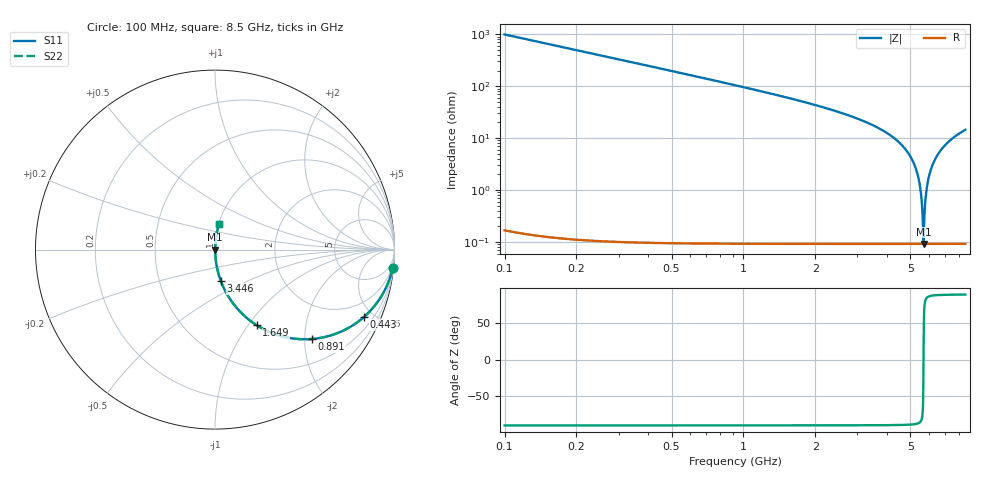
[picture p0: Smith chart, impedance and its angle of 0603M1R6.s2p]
! Created Wed Apr 18 13:49:44 2012
# hz S ma R 50
! 2 Port Network Data from SP1.SP block
! freq  magS11  angS11  magS21  angS21  magS12  angS12  magS22  angS22
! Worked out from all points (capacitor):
!   8401 points, 100 MHz to 8.5 GHz, reference 50 ohm
!   read as one part in series: C = 1.61 pF near 142 MHz
!   lowest |Z| = 92 mohm at 5.677 GHz (marker M1)
!   series resonance near 5.677 GHz, so ESL is about 490 pH
!   S11 on the Smith chart (normalised r, x): 100 MHz: 1, -20; 443 MHz: 1.00, -4.44; 891 MHz: 1.00, -2.16; 1.649 GHz: 1.00, -1.10; 3.446 GHz: 1.00, -0.36; 8.5 GHz: 1.00, +0.29
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1e8  0.9949 -5.8  0.1007 84.2  0.1007 84.2  0.9949 -5.8
2.49e8  0.9695 -14.2  0.2447 75.8  0.2447 75.8  0.9695 -14.2
4.43e8  0.9115 -24.3  0.411 65.7  0.411 65.7  0.9115 -24.3
8.91e8  0.7341 -42.7  0.6784 47.2  0.6784 47.2  0.7341 -42.7
1.5e9  0.5223 -58.4  0.852 31.5  0.852 31.5  0.5223 -58.4
1.649e9  0.4809 -61.2  0.876 28.7  0.876 28.7  0.4809 -61.2
2.9e9  0.2441 -75.7  0.9689 14.1  0.9689 14.1  0.2441 -75.7
3.446e9  0.1781 -79.4  0.9831 10.3  0.9831 10.3  0.1781 -79.4
4.3e9  0.09747 -83.9  0.9943 5.6  0.9943 5.6  0.09747 -83.9
4.933e9  0.04899 -86.1  0.9979 2.8  0.9979 2.8  0.04899 -86.1
5.331e9  0.02189 -86.3  0.9988 1.3  0.9988 1.3  0.02189 -86.3
5.541e9  0.008464 -83.3  0.999 0.5  0.999 0.5  0.008464 -83.3
5.599e9  0.004875 -78.9  0.9991 0.3  0.9991 0.3  0.004875 -78.9
5.653e9  0.001713 -57.5  0.9991 0.1  0.9991 0.1  0.001713 -57.5
5.677e9  0.0009188 1.8  0.9991 -0.0  0.9991 -0.0  0.0009188 1.8
5.7e9  0.001706 57.3  0.9991 -0.1  0.9991 -0.1  0.001706 57.3
5.755e9  0.004869 78.9  0.9991 -0.3  0.9991 -0.3  0.004869 78.9
5.814e9  0.008385 83.2  0.999 -0.5  0.999 -0.5  0.008385 83.2
6.038e9  0.02153 86.3  0.9989 -1.2  0.9989 -1.2  0.02153 86.3
6.45e9  0.04458 86.3  0.9981 -2.6  0.9981 -2.6  0.04458 86.3
7.1e9  0.07837 84.8  0.996 -4.5  0.996 -4.5  0.07837 84.8
8.5e9  0.1431 81.4  0.9888 -8.2  0.9888 -8.2  0.1431 81.4
